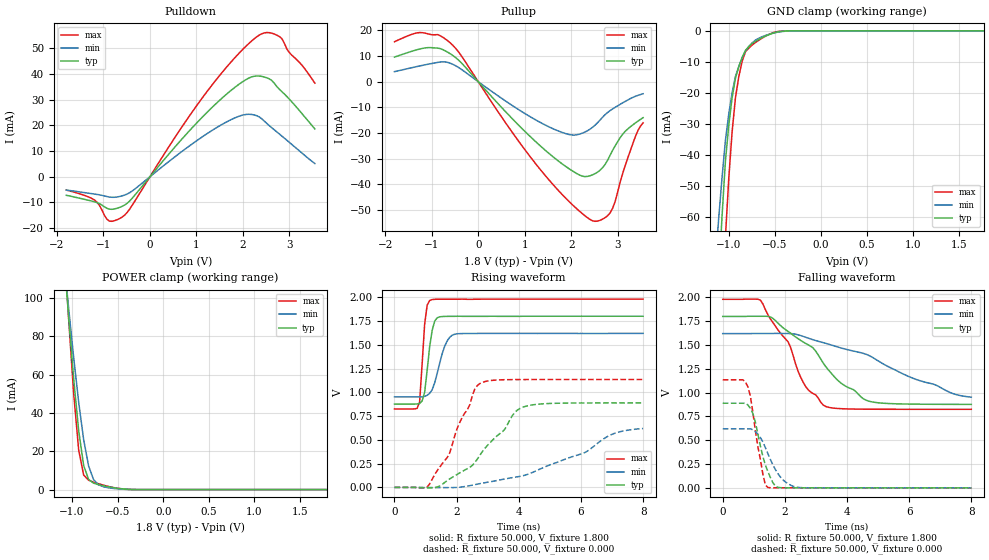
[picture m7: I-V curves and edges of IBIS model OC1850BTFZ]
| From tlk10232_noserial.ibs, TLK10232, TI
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[Model]   OC1850BTFZ
Model_type   3-state
Polarity   Non-Inverting
Enable   Active-Low
Cref =  15.0000pF
Rref =  100.0000M
Vref =  0V
Vmeas =  0.9
C_comp   1.025172p   0.8279542p   1.298979p
[Temperature Range]   25   125   -40
[Voltage Range]   1.8   1.62   1.98
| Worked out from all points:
|   slope of the pulldown table from 0 to 0.27 V, typ, clamps not added: 45.7 ohm
|   slope of the pullup table from 0 to 0.27 V, typ, clamps not added: 49.4 ohm
|   GND clamp passes 1 mA (typ) near -0.54 V on its own axis
|   POWER clamp passes 1 mA (typ) near -0.54 V on its own axis
|   rising waveform, R_fixture 50.000, V_fixture 1.800: 20-80 % time 204ps typ, 341ps min, 143ps max; typ from 0.877 V to 1.8 V
|   rising waveform, R_fixture 50.000, V_fixture 0.000: 20-80 % time 1.48ns typ, 2.52ns min, 970ps max; typ from 0 V to 0.889 V
|   falling waveform, R_fixture 50.000, V_fixture 1.800: 20-80 % time 1.77ns typ, 3.17ns min, 1.1ns max; typ from 1.8 V to 0.877 V
|   falling waveform, R_fixture 50.000, V_fixture 0.000: 20-80 % time 415ps typ, 565ps min, 333ps max; typ from 0.889 V to 0 V
[POWER_clamp]
-1.8V     626.5mA    508.8mA    755.8mA
-1.055V   100.8mA    103.1mA    102.4mA
-1.036V   89.33mA    94.12mA    88.27mA
-981.8mV  57.65mA    68.73mA    49.97mA
-927.3mV  30.72mA    45.57mA    20.64mA
-872.7mV  12.58mA    26.06mA    7.613mA
-818.2mV  5.289mA    12.28mA    4.901mA
-763.6mV  3.367mA    5.193mA    3.888mA
-709.1mV  2.574mA    2.507mA    3.06mA
-654.5mV  1.98mA     1.476mA    2.307mA
-436.4mV  343.9uA    170.5uA    303.6uA
1.8V      143.8nA    121.3nA    204.6nA
[Pulldown]
-1.8V     -7.226mA   -5.191mA   -5.197mA
-1.2V     -9.73mA    -6.722mA   -8.984mA
-872.7mV  -12.61mA   -7.901mA   -17.27mA
-545.5mV  -11.02mA   -7.145mA   -14.95mA
763.6mV   16.19mA    10.86mA    21.42mA
1.582V    31.1mA     20.68mA    41.25mA
2.073V    37.87mA    24.25mA    50.93mA
2.4V      39.06mA    22.61mA    55.6mA
2.618V    37.48mA    19.08mA    55.87mA
2.836V    33.12mA    15.81mA    53.75mA
3V        30.13mA    13.33mA    48.25mA
3.545V    18.59mA    5.139mA    36.44mA
[Pullup]
-1.8V     9.588mA    3.896mA    15.57mA
-1.255V   12.74mA    6.138mA    19.14mA
-872.7mV  13.08mA    7.495mA    18.35mA
-600mV    10.87mA    7.175mA    15.09mA
872.7mV   -17.04mA   -10.95mA   -23.32mA
1.582V    -28.9mA    -18.15mA   -39.58mA
2.073V    -35.35mA   -20.84mA   -48.82mA
2.455V    -36.38mA   -17.87mA   -54.24mA
2.673V    -33.6mA    -13.91mA   -53.65mA
2.891V    -26.78mA   -10.63mA   -49.37mA
3.327V    -16.83mA   -6.129mA   -24.05mA
3.545V    -14.04mA   -4.728mA   -16.08mA
[GND_clamp]
-1.8V     -597.6mA   -415.2mA   -913.8mA
-1.145V   -101.4mA   -74.85mA   -162.5mA
-1.109V   -79.51mA   -60.41mA   -127.5mA
-1.073V   -59.73mA   -47.23mA   -95.54mA
-1.036V   -42.01mA   -35.32mA   -66.57mA
-963.6mV  -21.55mA   -19.93mA   -32.55mA
-927.3mV  -15.28mA   -14.68mA   -21.5mA
-890.9mV  -11.53mA   -11.44mA   -14.72mA
-818.2mV  -6.261mA   -6.516mA   -6.7mA
-709.1mV  -3.317mA   -2.945mA   -3.729mA
-418.2mV  -133.1uA   -214.2uA   -64.17uA
1.764V    130.9nA    589.6nA    130.8nA
[Ramp]
dV/dt_f  0.5550065/1.775168n   0.3869261/3.184789n   0.6941227/1.100993n
dV/dt_r  0.5352009/1.497042n   0.3619876/2.539088n   0.6835905/0.9784663n
R_load = 50
[Rising Waveform]
R_fixture = 50.000
V_fixture = 1.800
V_fixture_min = 1.620
V_fixture_max = 1.980
|  time   V(typ)   V(min)   V(max)
0s        876.6mV    952.2mV    825mV
808.1ps   882.6mV    952.8mV    897.9mV
969.7ps   1V         957.5mV    1.714V
1.051ns   1.229V     969.1mV    1.916V
1.131ns   1.477V     989mV      1.965V
1.212ns   1.651V     1.027V     1.976V
1.374ns   1.784V     1.2V       1.979V
1.616ns   1.798V     1.485V     1.979V
1.939ns   1.799V     1.611V     1.979V
8ns       1.8V       1.62V      1.98V
[Rising Waveform]
R_fixture = 50.000
V_fixture = 0.000
V_fixture_min = 0.000
V_fixture_max = 0.000
|  time   V(typ)   V(min)   V(max)
0s        525.9nV    -2.92uV    623.9nV
1.051ns   -3.144mV   -1.875mV   3.498mV
1.778ns   89.78mV    -1.922mV   363.6mV
2.02ns    137.2mV    272.6uV    622.8mV
2.586ns   261.3mV    29.2mV     1.035V
2.828ns   376.9mV    44.87mV    1.104V
4.202ns   851.5mV    128.9mV    1.134V
6.141ns   888.1mV    369.4mV    1.135V
7.03ns    888.6mV    562.5mV    1.135V
8ns       888.7mV    619.7mV    1.135V
[Falling Waveform]
R_fixture = 50.000
V_fixture = 1.800
V_fixture_min = 1.620
V_fixture_max = 1.980
|  time   V(typ)   V(min)   V(max)
0s        1.8V       1.62V      1.98V
1.212ns   1.802V     1.621V     1.971V
1.535ns   1.795V     1.621V     1.773V
2.101ns   1.643V     1.621V     1.535V
2.667ns   1.517V     1.582V     1.064V
3.313ns   1.274V     1.518V     855.2mV
3.798ns   1.102V     1.47V      831.7mV
4.687ns   912.1mV    1.393V     826mV
6.061ns   879.6mV    1.159V     825mV
8ns       876.8mV    952.8mV    825mV
[Falling Waveform]
R_fixture = 50.000
V_fixture = 0.000
V_fixture_min = 0.000
V_fixture_max = 0.000
|  time   V(typ)   V(min)   V(max)
0s        888.7mV    620.2mV    1.135V
646.5ps   888.6mV    620.2mV    1.135V
808.1ps   871.1mV    620.1mV    1.062V
969.7ps   781.4mV    609.8mV    794.5mV
1.293ns   328.6mV    481.3mV    142.1mV
1.374ns   238.1mV    421.6mV    29.04mV
1.455ns   171mV      358.1mV    3.76mV
1.697ns   18.41mV    191.6mV    554uV
2.343ns   320.2uV    9.435mV    734.5uV
8ns       8.663uV    314.1uV    721.2nV
